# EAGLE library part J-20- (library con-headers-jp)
HEADER JACK PINS
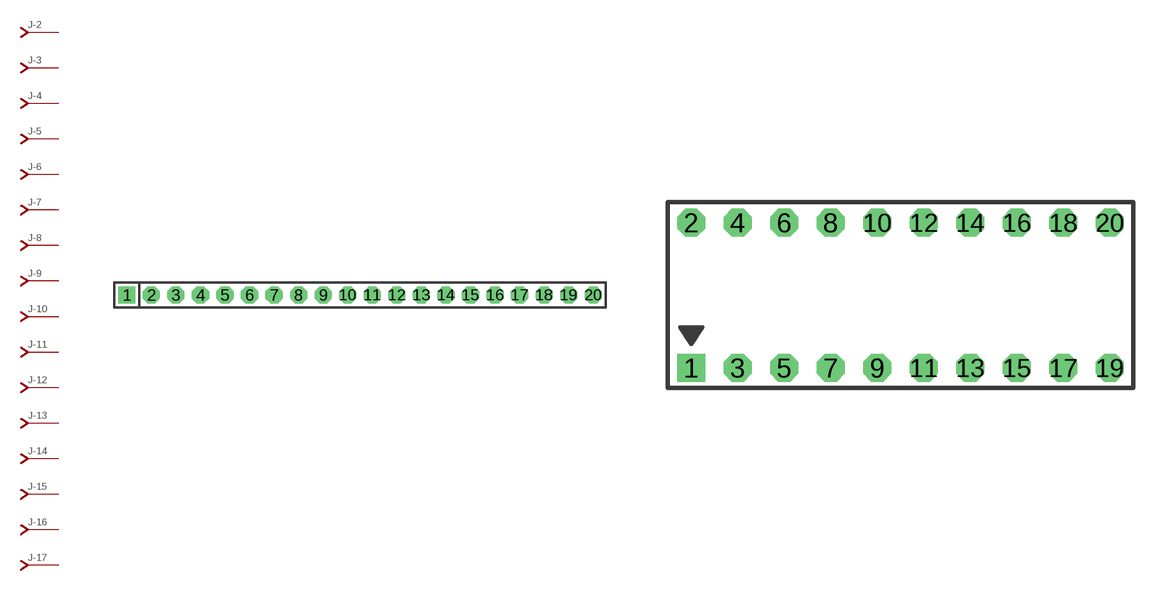
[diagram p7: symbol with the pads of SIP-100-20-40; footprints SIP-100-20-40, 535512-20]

Designator prefix J; gates -2=J-N -3=J-N -4=J-N -5=J-N -6=J-N -7=J-N -8=J-N -9=J-N -10=J-N -11=J-N -12=J-N -13=J-N -14=J-N -15=J-N -16=J-N -17=J-N -18=J-N -19=J-N -20=J-N -1=J-NV

## J-20-SIP-100-40  [SIP-100-20-40]
1  -1:J  pas
2  -2:J  pas
3  -3:J  pas
4  -4:J  pas
5  -5:J  pas
6  -6:J  pas
7  -7:J  pas
8  -8:J  pas
9  -9:J  pas
10  -10:J  pas
11  -11:J  pas
12  -12:J  pas
13  -13:J  pas
14  -14:J  pas
15  -15:J  pas
16  -16:J  pas
17  -17:J  pas
18  -18:J  pas
19  -19:J  pas
20  -20:J  pas

## J-20-535512  [535512-20]
Pads as for SIP-100-20-40

## J-20-79107  [79107-20]
Pads as for SIP-100-20-40

## J-20-79109  [79109-20]
Pads as for SIP-100-20-40

## J-20-87264  [87264-20]
Pads as for SIP-100-20-40

## J-20-87340  [87340-20]
Pads as for SIP-100-20-40

## J-20-87368  [87368-20]
Pads as for SIP-100-20-40

## J-20-100-2X10  [DIL-100-2X10]
Pads as for SIP-100-20-40

## J-20-100-2X10_M  [DIL-100-2X10_M]
Pads as for SIP-100-20-40

## J-20-2MM-2X10  [DIL-2MM-2X10]
Pads as for SIP-100-20-40

## J-20-2MM-2X10_M  [DIL-2MM-2X10_M]
Pads as for SIP-100-20-40

## J-20-SIP-100-32  [SIP-100-20-32]
Pads as for SIP-100-20-40

## J-20-SIP-100-40Y  [SIP-100-20-40Y]
Pads as for SIP-100-20-40

## J-20-SIP-100-32Y  [SIP-100-20-32Y]
Pads as for SIP-100-20-40

## J-20-71991  [79107-20]
Pads as for SIP-100-20-40

## J-20-KK-4455-B20  [KK-4455-B20]
Pads as for SIP-100-20-40

## J-20-KK-4455-A20  [KK-4455-A20]
Pads as for SIP-100-20-40

## J-20-KK-4455-C20  [KK-4455-C20]
Pads as for SIP-100-20-40

## Footprint SIP-100-20-40 (pad centres in mm)
SIP Header - 0.1", 40 mil drill
drill 1.016 pad 1.778 square: 1 -24.13,0
drill 1.016 pad 1.778 octagon: 2 -21.59,0; 3 -19.05,0; 4 -16.51,0; 5 -13.97,0; 6 -11.43,0; 7 -8.89,0; 8 -6.35,0; 9 -3.81,0; 10 -1.27,0; 11 1.27,0; 12 3.81,0; 13 6.35,0; 14 8.89,0; 15 11.43,0; 16 13.97,0; 17 16.51,0; 18 19.05,0; 19 21.59,0; 20 24.13,0

## Footprint 535512-20 (pad centres in mm)
AMPMODU - 535512 Series
drill 1.016 square: 1 -11.43,0
drill 1.016 octagon: 2 -11.43,7.938; 3 -8.89,0; 4 -8.89,7.938; 5 -6.35,0; 6 -6.35,7.938; 7 -3.81,0; 8 -3.81,7.938; 9 -1.27,0; 10 -1.27,7.938; 11 1.27,0; 12 1.27,7.938; 13 3.81,0; 14 3.81,7.938; 15 6.35,0; 16 6.35,7.938; 17 8.89,0; 18 8.89,7.938; 19 11.43,0; 20 11.43,7.938

## Footprint 79107-20 (pad centres in mm)
Molex Board-To-Board Receptacal 2.00mm (.079") Pitch Milli-Grid Header, Vertical, Through-Hole Mates with: 87759, 87762, 87758, 87760
drill 0.711 square: 1 -9,-1
drill 0.711: 2 -9,1; 3 -7,-1; 4 -7,1; 5 -5,-1; 6 -5,1; 7 -3,-1; 8 -3,1; 9 -1,-1; 10 -1,1; 11 1,-1; 12 1,1; 13 3,-1; 14 3,1; 15 5,-1; 16 5,1; 17 7,-1; 18 7,1; 19 9,-1; 20 9,1

## Footprint 79109-20 (pad centres in mm)
Molex Board-to-Board Receptacal 2.00mm (.079") Pitch Milli-Grid Header, Vertical, Top/Bottom Entry Mates with: 87758, 87759, 87760, 87831, 87832, 87833
smd 1.12 x 1.83: 1 -9,-2.65; 2 -9,2.65; 3 -7,-2.65; 4 -7,2.65; 5 -5,-2.65; 6 -5,2.65; 7 -3,-2.65; 8 -3,2.65; 9 -1,-2.65; 10 -1,2.65; 11 1,-2.65; 12 1,2.65; 13 3,-2.65; 14 3,2.65; 15 5,-2.65; 16 5,2.65; 17 7,-2.65; 18 7,2.65; 19 9,-2.65; 20 9,2.65
hole 0.914 at -8,0
hole 0.914 at -9,1
hole 0.914 at -9,-1
hole 0.914 at -7,-1
hole 0.914 at -7,1
hole 0.914 at -5,-1
hole 0.914 at -5,1
hole 0.914 at 8,0
hole 0.914 at -3,1
hole 0.914 at -3,-1
hole 0.914 at -1,1
hole 0.914 at -1,-1
hole 0.914 at 1,1
hole 0.914 at 1,-1
hole 0.914 at 3,1
hole 0.914 at 3,-1
hole 0.914 at 5,-1
hole 0.914 at 5,1
hole 0.914 at 7,1
hole 0.914 at 7,-1
hole 0.914 at 9,1
hole 0.914 at 9,-1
